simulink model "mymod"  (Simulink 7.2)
settings: Solver=ode45  StartTime=0.0  StopTime=10  FixedStep=.05  RelTol=1e-7
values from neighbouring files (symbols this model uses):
  q = 1    [second_init.m]
  w0 = 1    [second_init.m]
  zeta = max(.001,zeta)    [myfcost.m]    (also in second_init.m = 0.3)

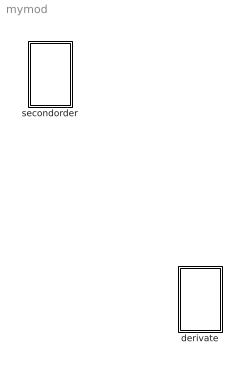
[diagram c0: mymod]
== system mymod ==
  derivate : Subsystem
  secondorder : Subsystem

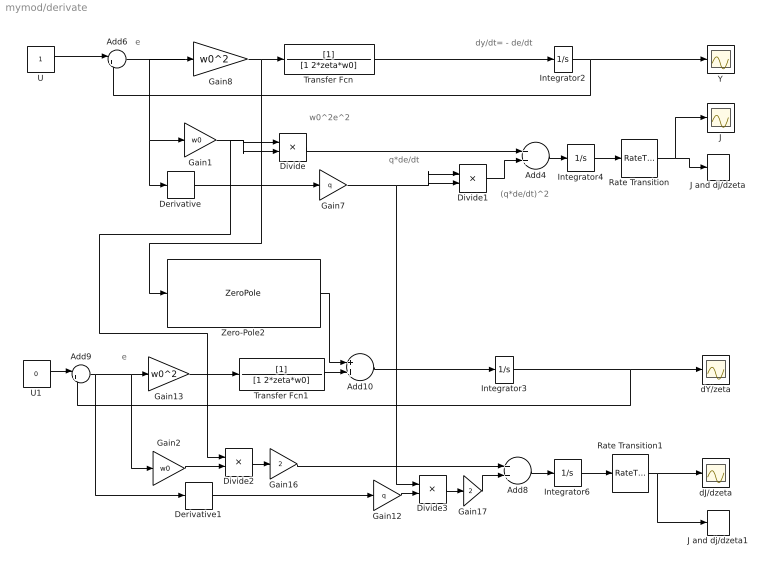
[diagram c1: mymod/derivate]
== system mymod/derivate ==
  note: e
  note: (q*de/dt)^2
  note: q*de/dt
  note: w0^2e^2
  note: dy/dt= - de/dt
  note: e
  Add10 : Sum  OutDataType=sfix(16)  OutScaling=2^-10
  Add4 : Sum  OutDataType=sfix(16)  OutScaling=2^-10
  Add6 : Sum  Inputs=|+-  OutDataType=sfix(16)  OutScaling=2^-10
  Add8 : Sum  OutDataType=sfix(16)  OutScaling=2^-10
  Add9 : Sum  Inputs=|+-  OutDataType=sfix(16)  OutScaling=2^-10
  Derivative : Derivative
  Derivative1 : Derivative
  Divide{,1..3} (4 alike) : Product  Inputs=**  OutDataType=sfix(16)  OutScaling=2^-10
  Gain1 : Gain  Gain=w0  ParameterDataType=sfix(16)  ParameterScaling=2^0  OutDataType=sfix(16)  OutScaling=2^0
  Gain12 : Gain  Gain=q  ParameterDataType=sfix(16)  ParameterScaling=2^0  OutDataType=sfix(16)  OutScaling=2^0
  Gain13 : Gain  Gain=w0^2  ParameterDataType=sfix(16)  ParameterScaling=2^0  OutDataType=sfix(16)  OutScaling=2^0
  Gain16 : Gain  Gain=2  ParameterDataType=sfix(16)  ParameterScaling=2^0  OutDataType=sfix(16)  OutScaling=2^0
  Gain17 : Gain  Gain=2  ParameterDataType=sfix(16)  ParameterScaling=2^0  OutDataType=sfix(16)  OutScaling=2^0
  Gain2 : Gain  Gain=w0  ParameterDataType=sfix(16)  ParameterScaling=2^0  OutDataType=sfix(16)  OutScaling=2^0
  Gain7 : Gain  Gain=q  ParameterDataType=sfix(16)  ParameterScaling=2^0  OutDataType=sfix(16)  OutScaling=2^0
  Gain8 : Gain  Gain=w0^2  ParameterDataType=sfix(16)  ParameterScaling=2^0  OutDataType=sfix(16)  OutScaling=2^0
  Integrator{2..4,6} (4 alike) : Integrator
  J : Scope
  J and dj/dzeta : ToWorkspace  VariableName=out  SampleTime=-1  SaveFormat=Array
  J and dj/dzeta1 : ToWorkspace  VariableName=dout  SampleTime=-1  SaveFormat=Array
  Rate Transition : RateTransition  OutPortSampleTime=Tsample
  Rate Transition1 : RateTransition  OutPortSampleTime=Tsample
  Transfer Fcn : TransferFcn  Denominator=[1 2*zeta*w0]
  Transfer Fcn1 : TransferFcn  Denominator=[1 2*zeta*w0]
  U : Constant  OutDataType=sfix(16)  OutScaling=2^0
  U1 : Constant  Value=0  OutDataType=sfix(16)  OutScaling=2^0
  Y : Scope
  Zero-Pole2 : ZeroPole  Zeros=[]  Poles=[-2*zeta*w0,-2*zeta*w0]  Gain=[-2*w0]
  dJ/dzeta : Scope
  dY/zeta : Scope
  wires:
  Integrator2/1 -> Add6/2, Y/1
  Gain17/1 -> Add8/2
  Gain16/1 -> Add8/1
  Zero-Pole2/1 -> Add10/1
  Transfer Fcn1/1 -> Add10/2
  Add10/1 -> Integrator3/1
  Add8/1 -> Integrator6/1
  Divide2/1 -> Gain16/1
  Gain13/1 -> Transfer Fcn1/1
  Integrator6/1 -> Rate Transition1/1
  Divide3/1 -> Gain17/1
  Gain12/1 -> Divide3/2
  U1/1 -> Add9/1
  Add9/1 -> Gain13/1, Gain2/1, Derivative1/1
  Add4/1 -> Integrator4/1
  Divide/1 -> Add4/1
  Gain8/1 -> Zero-Pole2/1, Transfer Fcn/1
  Integrator4/1 -> Rate Transition/1
  Transfer Fcn/1 -> Integrator2/1
  Divide1/1 -> Add4/2
  Gain7/1 -> Divide3/1, Divide1/1, Divide1/2
  Add6/1 -> Gain8/1, Derivative/1, Gain1/1
  Gain1/1 -> Divide/1, Divide/2, Divide2/1
  Derivative/1 -> Gain7/1
  Gain2/1 -> Divide2/2
  Derivative1/1 -> Gain12/1
  Integrator3/1 -> Add9/2, dY/zeta/1
  U/1 -> Add6/1
  Rate Transition/1 -> J/1, J and dj/dzeta/1
  Rate Transition1/1 -> dJ/dzeta/1, J and dj/dzeta1/1

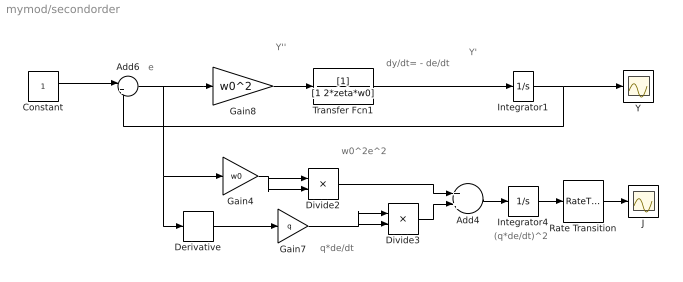
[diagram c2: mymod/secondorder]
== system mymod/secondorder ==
  note: (q*de/dt)^2
  note: q*de/dt
  note: w0^2e^2
  note: dy/dt= - de/dt
  note: e
  note: Y''
  note: Y'
  Add4 : Sum  OutDataType=sfix(16)  OutScaling=2^-10
  Add6 : Sum  Inputs=|+-  OutDataType=sfix(16)  OutScaling=2^-10
  Constant : Constant  OutDataType=sfix(16)  OutScaling=2^0
  Derivative : Derivative
  Divide2 : Product  Inputs=**  OutDataType=sfix(16)  OutScaling=2^-10
  Divide3 : Product  Inputs=**  OutDataType=sfix(16)  OutScaling=2^-10
  Gain4 : Gain  Gain=w0  ParameterDataType=sfix(16)  ParameterScaling=2^0  OutDataType=sfix(16)  OutScaling=2^0
  Gain7 : Gain  Gain=q  ParameterDataType=sfix(16)  ParameterScaling=2^0  OutDataType=sfix(16)  OutScaling=2^0
  Gain8 : Gain  Gain=w0^2  ParameterDataType=sfix(16)  ParameterScaling=2^0  OutDataType=sfix(16)  OutScaling=2^0
  Integrator1 : Integrator
  Integrator4 : Integrator
  J : Scope
  Rate Transition : RateTransition  OutPortSampleTime=Tsample
  Transfer Fcn1 : TransferFcn  Denominator=[1 2*zeta*w0]
  Y : Scope
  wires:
  Integrator1/1 -> Add6/2, Y/1
  Add4/1 -> Integrator4/1
  Divide2/1 -> Add4/1
  Gain8/1 -> Transfer Fcn1/1
  Transfer Fcn1/1 -> Integrator1/1
  Divide3/1 -> Add4/2
  Gain7/1 -> Divide3/1, Divide3/2
  Add6/1 -> Gain8/1, Derivative/1, Gain4/1
  Gain4/1 -> Divide2/1, Divide2/2
  Derivative/1 -> Gain7/1
  Constant/1 -> Add6/1
  Rate Transition/1 -> J/1
  Integrator4/1 -> Rate Transition/1
